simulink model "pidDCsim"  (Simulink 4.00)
settings: Solver=ode45  SolverMode=SingleTasking  StartTime=0.0  StopTime=50  RelTol=1e-3  AbsTol=1e-6
libraries: simulink3 x1, adaptlib x1

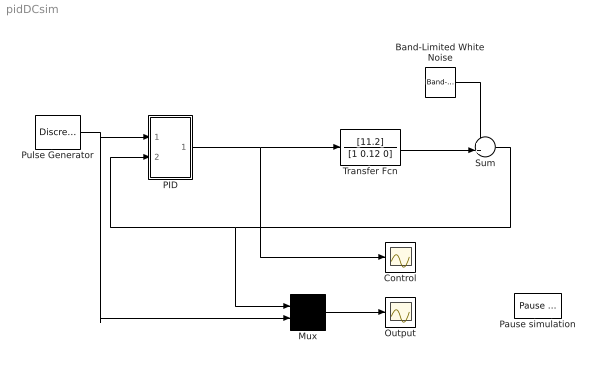
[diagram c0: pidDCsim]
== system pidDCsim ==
  Band-Limited White Noise : simulink3/Sources/Band-Limited White Noise  Cov=[0.00001]  Ts=0.1  seed=[23341]
  Control : Scope
  Mux : Mux  Inputs=2
  Output : Scope
  PID : Subsystem  mask{K=1.7, Ti=1.25, Td=0.3}
      mask init:
      | b_reg=1; c_reg=0; Ts=0.01;
  Pause simulation : adaptlib/Pause simulation  par=[25]
  Pulse Generator : DiscretePulseGenerator  PulseType=Time-based  Amplitude=2  Period=10  PulseWidth=50  PhaseDelay=0  SampleTime=1
  Sum : Sum  Inputs=++|  SaturateOnIntegerOverflow=on
  Transfer Fcn : TransferFcn  Numerator=[11.2]  Denominator=[1 0.12 0]  AbsoluteTolerance=auto  Realization=auto
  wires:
  Mux/1 -> Output/1
  Pulse Generator/1 -> Mux/2, PID/1(uc)
  PID/1(Out1) -> Control/1, Transfer Fcn/1
  Transfer Fcn/1 -> Sum/2
  Sum/1 -> Mux/1, PID/2(y)
  Band-Limited White Noise/1 -> Sum/1

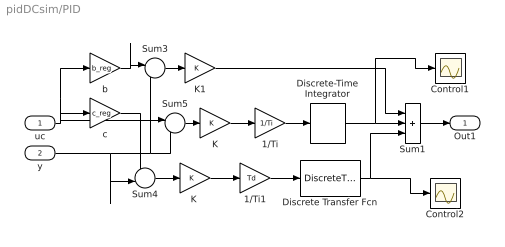
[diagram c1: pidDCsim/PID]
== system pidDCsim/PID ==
  uc : Inport  Port=1  LatchInput=off
  y : Inport  Port=2  LatchInput=off
  1/Ti : Gain  Gain=1/Ti  Multiplication=Element-wise(K.*u)  SaturateOnIntegerOverflow=on
  1/Ti1 : Gain  Gain=Td  Multiplication=Element-wise(K.*u)  SaturateOnIntegerOverflow=on
  Control1 : Scope
  Control2 : Scope
  Discrete Transfer Fcn : DiscreteTransferFcn  Numerator=[1 -1]*1/(Td/10+Ts)  Denominator=[1 -Td/(Td+10*Ts)]  SampleTime=Ts  Realization=auto
  Discrete-Time Integrator : DiscreteIntegrator  IntegratorMethod=ForwardEuler  ExternalReset=none  InitialConditionSource=internal  InitialCondition=0  LimitOutput=off  UpperSaturationLimit=inf  LowerSaturationLimit=-inf  ShowSaturationPort=off  ShowStatePort=off  SampleTime=Ts
  K : Gain  Gain=K  Multiplication=Element-wise(K.*u)  SaturateOnIntegerOverflow=on
  "K " : Gain  Gain=K  Multiplication=Element-wise(K.*u)  SaturateOnIntegerOverflow=on
  K1 : Gain  Gain=K  Multiplication=Element-wise(K.*u)  SaturateOnIntegerOverflow=on
  Sum1 : Sum  Inputs=+++  SaturateOnIntegerOverflow=on
  Sum3 : Sum  Inputs=+-  SaturateOnIntegerOverflow=on
  Sum4 : Sum  Inputs=+-  SaturateOnIntegerOverflow=on
  Sum5 : Sum  Inputs=+-  SaturateOnIntegerOverflow=on
  b : Gain  Gain=b_reg  Multiplication=Element-wise(K.*u)  SaturateOnIntegerOverflow=on
  c : Gain  Gain=c_reg  Multiplication=Element-wise(K.*u)  SaturateOnIntegerOverflow=on
  Out1 : Outport  Port=1
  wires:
  Sum5/1 -> K/1
  Sum4/1 -> "K "/1
  c/1 -> Sum4/1
  K1/1 -> Sum1/1
  Sum3/1 -> K1/1
  y/1 -> Sum5/2, Sum3/2, Sum4/2
  b/1 -> Sum3/1
  uc/1 -> Sum5/1, b/1, c/1
  "K "/1 -> 1/Ti1/1
  1/Ti1/1 -> Discrete Transfer Fcn/1
  Discrete Transfer Fcn/1 -> Control2/1, Sum1/3
  Discrete-Time Integrator/1 -> Control1/1, Sum1/2
  Sum1/1 -> Out1/1
  1/Ti/1 -> Discrete-Time Integrator/1
  K/1 -> 1/Ti/1
